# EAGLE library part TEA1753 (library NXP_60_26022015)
The GreenChip III is the third generation of green Switched Mode Power Supply (SMPS) controller ICs. The GreenChip III combines a controller for Power Factor Correction (PFC) and a flyback controller. Its high level of integration allows the design of a cost-effective power supply with a very low number of external components. AAL Eindhoven MK
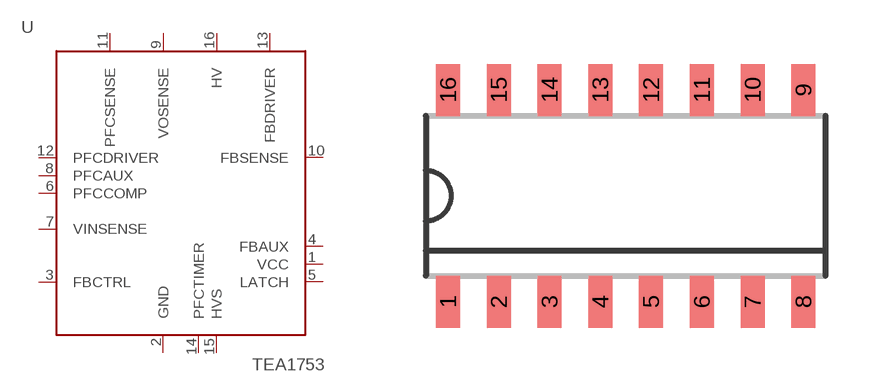
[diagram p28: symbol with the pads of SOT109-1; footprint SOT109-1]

Designator prefix U

## TEA1753T (12NC: 9352 932 05518)  [SOT109-1]
1  VCC
2  GND
3  FBCTRL
4  FBAUX
5  LATCH
6  PFCCOMP
7  VINSENSE
8  PFCAUX
9  VOSENSE
10  FBSENSE
11  PFCSENSE
12  PFCDRIVER
13  FBDRIVER
14  PFCTIMER
15  HVS
16  HV

## Footprint SOT109-1 (pad centres in mm)
SOT109-1 SO16: plastic small outline package; 16 leads; body width 3.9 mm JEDEC: MS-012 IEC: 076E07
smd 0.6 x 1.3: 1 -4.445,-2.65; 2 -3.175,-2.65; 3 -1.905,-2.65; 4 -0.635,-2.65; 5 0.635,-2.65; 6 1.905,-2.65; 7 3.175,-2.65; 8 4.445,-2.65; 9 4.445,2.65; 10 3.175,2.65; 11 1.905,2.65; 12 0.635,2.65; 13 -0.635,2.65; 14 -1.905,2.65; 15 -3.175,2.65; 16 -4.445,2.65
